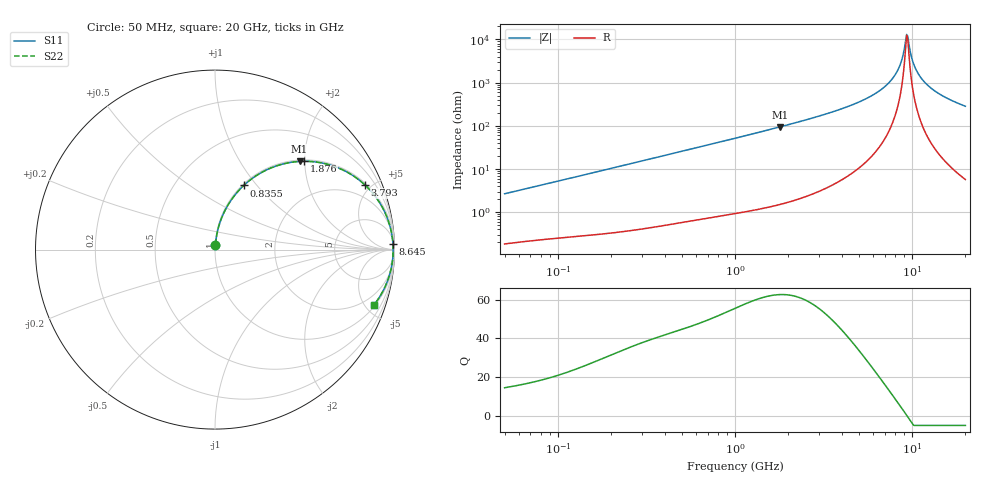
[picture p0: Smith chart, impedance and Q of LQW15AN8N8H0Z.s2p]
!Murata Part Number: LQW15AN8N8H0Z
!These Parameters are Measured in Series Mode Connection
!  o--[Z]--o
!Port1  Port2
!  o-------o
!Freq. Start=50[MHz] Stop=20[GHz], 401[Steps]
# Hz S RI R 50
!Freq.(Hz) S11(Real) S11(Imag) S21(Real) S21(Imag) S12(Real) S12(Imag) S22(Real) S22(Imag)
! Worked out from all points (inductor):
!   401 points, 50 MHz to 20 GHz, reference 50 ohm
!   read as one part in series: L = 8.42 nH near 51.52 MHz
!   highest Q = 62.5 at 1.793 GHz (marker M1), where L = 8.37 nH
!   self-resonance near 9.317 GHz
!   S11 on the Smith chart (normalised r, x): 50 MHz: 1.00, +0.05; 835.5 MHz: 1.02, +0.86; 1.876 GHz: 1.03, +1.98; 3.793 GHz: 1.10, +4.59; 8.645 GHz: 13, +56; 20 GHz: 1.11, -5.68
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5e7  0.00254 0.0265  0.9975 -0.0265  0.9975 -0.0265  0.00254 0.0265
1.364002e8  0.00777 0.0702  0.9922 -0.0702  0.9922 -0.0702  0.00777 0.0702
3.721004e8  0.0396 0.183  0.9604 -0.183  0.9604 -0.183  0.0396 0.183
8.354841e8  0.1601 0.3572  0.8399 -0.3572  0.8399 -0.3572  0.1601 0.3572
1e9  0.2134 0.4008  0.7866 -0.4008  0.7866 -0.4008  0.2134 0.4008
1.793498e9  0.4713 0.4912  0.5287 -0.4912  0.5287 -0.4912  0.4713 0.4912
1.875929e9  0.4951 0.492  0.5049 -0.492  0.5049 -0.492  0.4951 0.492
2.728004e9  0.6917 0.4532  0.3083 -0.4532  0.3083 -0.4532  0.6917 0.4532
3.792786e9  0.8352 0.3605  0.1648 -0.3605  0.1648 -0.3605  0.8352 0.3605
5.683258e9  0.947 0.2064  0.053 -0.2064  0.053 -0.2064  0.947 0.2064
7.442007e9  0.9832 0.0955  0.0168 -0.0955  0.0168 -0.0955  0.9832 0.0955
8.141811e9  0.9891 0.0582  0.0109 -0.0582  0.0109 -0.0582  0.9891 0.0582
8.644534e9  0.9915 0.0332  0.00851 -0.0332  0.00851 -0.0332  0.9915 0.0332
9.178299e9  0.9926 0.00832  0.00742 -0.00832  0.00742 -0.00832  0.9926 0.00832
9.457416e9  0.9927 -0.00415  0.00734 0.00415  0.00734 0.00415  0.9927 -0.00415
9.600142e9  0.9926 -0.0104  0.00742 0.0104  0.00742 0.0104  0.9926 -0.0104
1.004137e10  0.9919 -0.0291  0.00813 0.0291  0.00813 0.0291  0.9919 -0.0291
1.034674e10  0.991 -0.0416  0.009 0.0416  0.009 0.0416  0.991 -0.0416
1.082228e10  0.9891 -0.0603  0.0109 0.0603  0.0109 0.0603  0.9891 -0.0603
1.166392e10  0.9843 -0.0914  0.0157 0.0914  0.0157 0.0914  0.9843 -0.0914
1.460232e10  0.9574 -0.1844  0.0426 0.1844  0.0426 0.1844  0.9574 -0.1844
2e10  0.8847 -0.3095  0.1153 0.3095  0.1153 0.3095  0.8847 -0.3095
